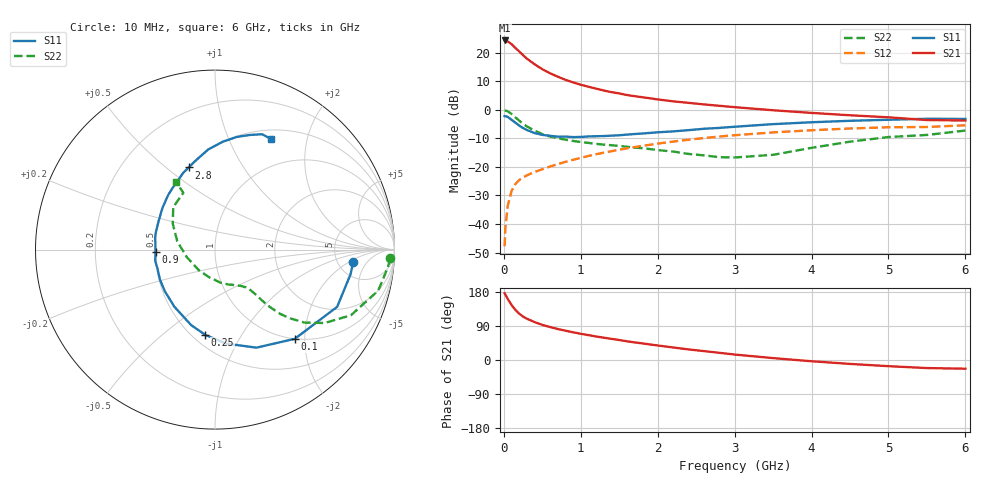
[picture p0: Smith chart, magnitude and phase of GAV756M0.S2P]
! Infineon Technologies  Discrete & RF Semiconductors
! BF775
! Si NPN RF Bipolar Junction Transistor in SOT23
! VCE = 0.75 V  IC = 6 mA
! Common Emitter S-Parameters:  May  1996
# GHz  S  MA  R  50
!  f  S11  S21  S12  S22
! GHz  MAG  ANG  MAG  ANG  MAG  ANG  MAG  ANG
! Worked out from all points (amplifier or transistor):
!   36 points, 10 MHz to 6 GHz, reference 50 ohm
!   highest |S21| = 24.2 dB at 10 MHz (marker M1)
!   |S21| within 3 dB of that: start of sweep to 165.4 MHz
!   unconditionally stable (mu >= 1): 614.2 MHz to end of sweep
!   at 250 MHz: K = 0.58, MSG = 21.4 dB, |S12| = -23.7 dB
!   at 1.4 GHz: K = 1.19, MAG = 7.7 dB, |S12| = -14.5 dB
!   at 6 GHz: K = 1.05, MAG = -0.5 dB, |S12| = -5.4 dB
!   S11 on the Smith chart (normalised r, x): 10 MHz: 6.91, -2.45; 100 MHz: 1.00, -1.79; 250 MHz: 0.58, -0.71; 900 MHz: 0.50, -0.01; 2.8 GHz: 0.51, +0.60; 6 GHz: 0.62, +1.45
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0.01  0.7726 -5.3  16.27 176.3  0.0041 86.2  0.9782 -2.9
0.02  0.7677 -10.3  15.97 172.2  0.0087 83.4  0.9684 -5.8
0.05  0.7516 -25.1  15.64 161.4  0.0206 77.0  0.9377 -14.1
0.1  0.6668 -48.2  14.05 145.3  0.0378 66.9  0.8409 -25.8
0.15  0.5931 -67.1  12.03 132.1  0.0502 60.0  0.7351 -33.8
0.2  0.5272 -83.3  10.44 122.3  0.0588 55.7  0.6428 -39.2
0.25  0.4778 -96.6  8.983 114.6  0.0653 52.8  0.5649 -42.6
0.3  0.4409 -107.6  7.828 108.9  0.0711 52.3  0.5097 -44.6
0.4  0.3902 -125.6  6.228 100.0  0.0815 51.5  0.4302 -46.6
0.5  0.3631 -140.3  5.108 92.7  0.0908 52.2  0.3748 -47.4
0.6  0.3493 -151.5  4.345 87.0  0.1013 52.8  0.3398 -47.8
0.7  0.3376 -161.5  3.784 81.8  0.1116 53.3  0.3172 -48.3
0.9  0.3317 -177.8  3.001 73.1  0.1329 53.8  0.2841 -49.5
1.1  0.3408 168.4  2.521 65.6  0.1551 53.8  0.2625 -52.3
1.3  0.3462 158.4  2.167 58.8  0.1774 52.8  0.2449 -55.3
1.6  0.367 144.4  1.807 49.4  0.2105 50.8  0.2247 -61.8
2.2  0.4176 124.3  1.401 33.1  0.2768 44.8  0.1855 -81.1
2.8  0.4803 107.6  1.171 19.0  0.3393 37.4  0.1479 -113.8
3.5  0.5591 93.9  0.978 5.0  0.4006 27.7  0.1625 -164.7
4.5  0.6396 79.0  0.799 -10.3  0.4694 14.2  0.2759 148.5
5.5  0.6944 67.8  0.659 -21.3  0.4983 0.8  0.3616 119.2
6  0.6907 62.9  0.647 -23.0  0.534 -3.0  0.432 119.8
